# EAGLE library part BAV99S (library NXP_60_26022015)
High-speed switching diode High-speed switching diodes, encapsulated in small Surface-Mounted Device (SMD) plastic packages. AAL Eindhoven MK
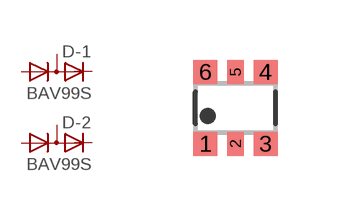
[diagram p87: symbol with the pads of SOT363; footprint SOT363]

Designator prefix D; gates -1=DIODE_AKAK -2=DIODE_AKAK

## BAV99S  [SOT363]
1  -1:A1  pas
2  -1:K2  pas
3  -2:K1A2  pas
4  -2:A1  pas
5  -2:K2  pas
6  -1:K1A2  pas

## Footprint SOT363 (pad centres in mm)
SOT363 Plastic surface-mounted package; 6 leads JEDEC: -- IEC: -- JEITA: SC-88
smd 0.6 x 0.6: 1 -0.75,-0.9; 3 0.75,-0.9; 4 0.75,0.9; 6 -0.75,0.9
smd 0.4 x 0.6: 2 0,-0.9; 5 0,0.9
